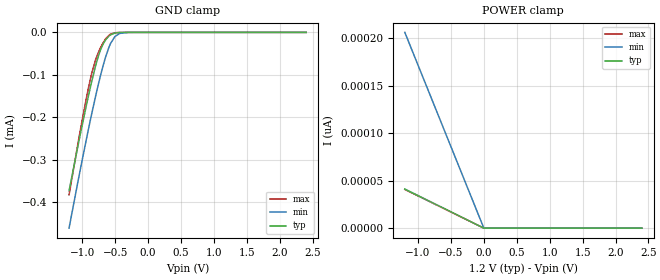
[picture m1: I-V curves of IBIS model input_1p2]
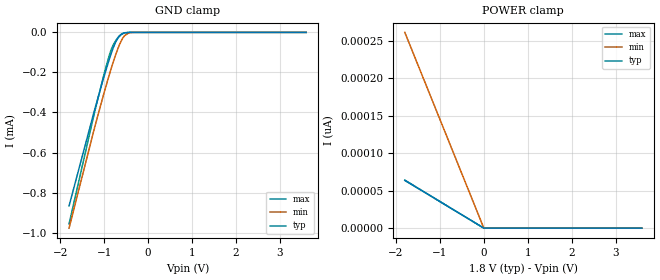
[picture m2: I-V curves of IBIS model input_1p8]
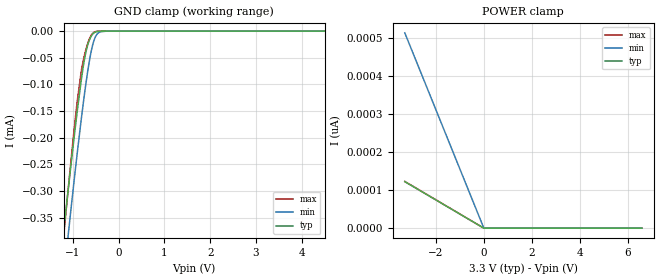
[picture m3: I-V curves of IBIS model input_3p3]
|Texas Instruments Incorporated
|TMUX1208 5-V General Purpose, Analog Multiplexer
[IBIS Ver]   4.1
[File name]   tmux1208.ibs
[Date]   09/12/2018
[File Rev]   1.0
[Source]
| Texas Instruments Incorporated.
| Analog-eLab Design Center, HPA
| 12500 TI Blvd
| Dallas, TX -75243
[Notes]   Revision History:
| Rev 1.0: 09/12/2018
| - Initial version of the model
| - Model generated from simulations in SPECTRE
| - Model names with a trailing _1p2 contain the model for 1.2V operation.
|   Model names with a trailing _1p8 contain the model for 1.8V operation.
|   Model names with a trailing _3p3 contain the model for 3.3V operation.
|   Model names with a trailing _5p0 contain the model for 5.0V operation.
| - C_comp although listed in numerical order of value are
|   obtained from varying PVT conditions. For PVT conditions for
|   each specific value refer the buffer description under
|   respective [Model]. IBIS model user is responsible for using
|   appropriate C_comp to simulate for Signal Integrity.
[Disclaimer]
| This model is designed as an aid for customers of Texas Instruments.
| TI and its licensors and suppliers make no warranties, either expressed
| or implied, with respect to this  model, including the warranties of
| merchantability or fitness for a particular purpose. The model is
| provided solely on an "as is" basis. The entire risk as to its quality
| and performance is with the customer.
| This model is subject to change without notice. Texas Instruments
| Incorporated is not responsible for updating this model.
[Copyright]
(C) Copyright 2018 Texas Instruments Incorporated.All rights reserved.
|  Component TMUX1208PW 16-pin TSSOP - PW package
|  Part # TMUX1208PW
[Component]   TMUX1208PW
[Manufacturer]  TI
[Package]   |16 TSSOP- PW package
|   typ   min   max
R_pkg   0.05   0.04   0.06
L_pkg   1.0nH   0.8nH   1.2nH
C_pkg   0.2pF   0.16pF   0.24pF
[Pin]  signal_name  model_name  R_pin   L_pin   C_pin
1   A0   input   NA   NA   NA
2   EN   input   NA   NA   NA
3   N.C.   nc   NA   NA   NA
4   S1   nc   NA   NA   NA
5   S2   nc   NA   NA   NA
6   S3   nc   NA   NA   NA
7   S4   nc   NA   NA   NA
8   D   nc   NA   NA   NA
9   S8   nc   NA   NA   NA
10   S7   nc   NA   NA   NA
11   S6   nc   NA   NA   NA
12   S5   nc   NA   NA   NA
13   VDD   power   NA   NA   NA
14   GND   gnd   NA   NA   NA
15   A2   input   NA   NA   NA
16   A1   input   NA   NA   NA
|  Component TMUX1208RSV 16-pin QFN - RSV package
|  Part # TMUX1208RSV
[Component]   TMUX1208RSV
[Manufacturer]  TI
[Package]   |16 QFN- RSV package
|   typ   min   max
R_pkg   0.05   0.04   0.06
L_pkg   1.0nH   0.8nH   1.2nH
C_pkg   0.2pF   0.16pF   0.24pF
[Pin]  signal_name   model_name  R_pin   L_pin   C_pin
1   N.C.   nc   NA   NA   NA
2   S1   nc   NA   NA   NA
3   S2   nc   NA   NA   NA
4   S3   nc   NA   NA   NA
5   S4   nc   NA   NA   NA
6   D   nc   NA   NA   NA
7   S8   nc   NA   NA   NA
8   S7   nc   NA   NA   NA
9   S6   nc   NA   NA   NA
10   S5   nc   NA   NA   NA
11   VDD   power   NA   NA   NA
12   GND   gnd   NA   NA   NA
13   A2   input   NA   NA   NA
14   A1   input   NA   NA   NA
15   A0   input   NA   NA   NA
16   EN   input   NA   NA   NA
|   Model Selectors
[Model Selector] input
input_1p2   1.2V   digital Input
input_1p8   1.8V   digital Input
input_3p3   3.3V   digital Input
input_5p0   5.0V   digital Input
| Models and submodels in the file (4): input_1p2 (Input), input_1p8 (Input), input_3p3 (Input), input_5p0 (Input)
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|   input_1p2 Model
[Model]   input_1p2
Model_type   Input
Vinl = 0.36
Vinh = 0.96
|   typ   min   max
C_comp   2.059E-15   2.021E-15   2.117E-15
| Where Nom  PVT is Nominal Process, 1.2V, 25C
|   Fast PVT is Strong Process,  1.32V, -40C
|   Slow PVT is Weak Process,   1.08V, 125C
[Voltage Range]   1.2   1.08   1.32
|Junction Temperature
[Temperature Range]   25   125   -40
[Power Clamp Reference]   1.2   1.08   1.32
[GND Clamp Reference]   0   0   0
[GND Clamp]
|   Voltage   I(typ)   I(min)   I(max)
-1.2V     -373uA     -460.8uA   -382.4uA
-1.02V    -233.2uA   -315.6uA   -222.8uA
-933.6mV  -169.4uA   -249uA     -152.2uA
-854.4mV  -114.7uA   -190.6uA   -95.31uA
-800.4mV  -80.84uA   -152.6uA   -66uA
-750mV    -53.72uA   -119.1uA   -45.8uA
-685.2mV  -28.28uA   -79.66uA   -25.23uA
-591.6mV  -8.354uA   -34.01uA   -6.608uA
-501.6mV  -1.595uA   -9.468uA   -936.7nA
-429.6mV  -317.5nA   -2.423uA   -127.1nA
-300mV    -9.022nA   -139.4nA   -695.2pA
2.4V      0A         0A         0A
[POWER Clamp]
|   Voltage   I(typ)   I(min)   I(max)
-1.2V     41.25pA    206.3pA    40.81pA
0V        0A         0A         0A
2.4V      0A         0A         0A
|   input_1p8 Model
[Model]   input_1p8
Model_type   Input
Vinl = 0.68
Vinh = 1.07
|   typ   min   max
C_comp   2.059E-15   2.021E-15   2.117E-15
| Where Nom  PVT is Nominal Process, 1.8V, 25C
|   Fast PVT is Strong Process,  1.98V, -40C
|   Slow PVT is Weak Process,   1.62V, 125C
[Voltage Range]   1.8   1.62   1.98
|Junction Temperature
[Temperature Range]   25   125   -40
[Power Clamp Reference]   1.8   1.62   1.98
[GND Clamp Reference]   0   0   0
[GND Clamp]
|   Voltage   I(typ)   I(min)   I(max)
-1.8V     -866.6uA   -977.4uA   -956.3uA
-1.244V   -407.9uA   -497.1uA   -422.8uA
-984.6mV  -206.7uA   -288uA     -193.2uA
-882mV    -133.2uA   -210.6uA   -113.7uA
-828mV    -97.66uA   -171.8uA   -79.76uA
-725.4mV  -42.71uA   -103.6uA   -37.35uA
-676.8mV  -25.79uA   -74.93uA   -22.98uA
-622.8mV  -13.23uA   -47.28uA   -11.18uA
-536.4mV  -3.191uA   -16.5uA    -2.139uA
-444.6mV  -452.6nA   -3.278uA   -199.2nA
-363.6mV  -57.98nA   -590.6nA   -13.44nA
3.6V      0A         0A         0A
[POWER Clamp]
|   Voltage   I(typ)   I(min)   I(max)
-1.8V     63.66pA    261.2pA    64.08pA
0V        0A         0A         0A
3.6V      0A         0A         0A
|   input_3p3 Model
[Model]   input_3p3
Model_type   Input
Vinl = 0.8
Vinh = 1.35
|   typ   min   max
C_comp   2.059E-15   2.021E-15   2.126E-15
| Where Nom  PVT is Nominal Process, 3.3V, 25C
|   Fast PVT is Strong Process,  3.63V, -40C
|   Slow PVT is Weak Process,   2.97V, 125C
[Voltage Range]   3.3   2.97   3.63
|Junction Temperature
[Temperature Range]   25   125   -40
[Power Clamp Reference]   3.3   2.97   3.63
[GND Clamp Reference]   0   0   0
[GND Clamp]
|   Voltage   I(typ)   I(min)   I(max)
-3.3V     -2.159mA   -2.35mA    -2.449mA
-1.211V   -381.8uA   -469.9uA   -392.6uA
-1.181V   -358.2uA   -445.4uA   -365.4uA
-1.102V   -296.1uA   -381uA     -294.2uA
-943.8mV  -176.8uA   -256.7uA   -160.2uA
-815.1mV  -89.66uA   -162.8uA   -73.02uA
-686.4mV  -28.65uA   -80.35uA   -25.56uA
-607.2mV  -10.59uA   -40.36uA   -8.685uA
-528mV    -2.713uA   -14.54uA   -1.765uA
-409.2mV  -190.8nA   -1.586uA   -65.52nA
-260.7mV  -645pA     -53.76nA   0A
6.6V      0A         0A         0A
[POWER Clamp]
|   Voltage   I(typ)   I(min)   I(max)
-3.3V     122.3pA    513.9pA    123.1pA
0V        0A         0A         0A
6.6V      0A         0A         0A
